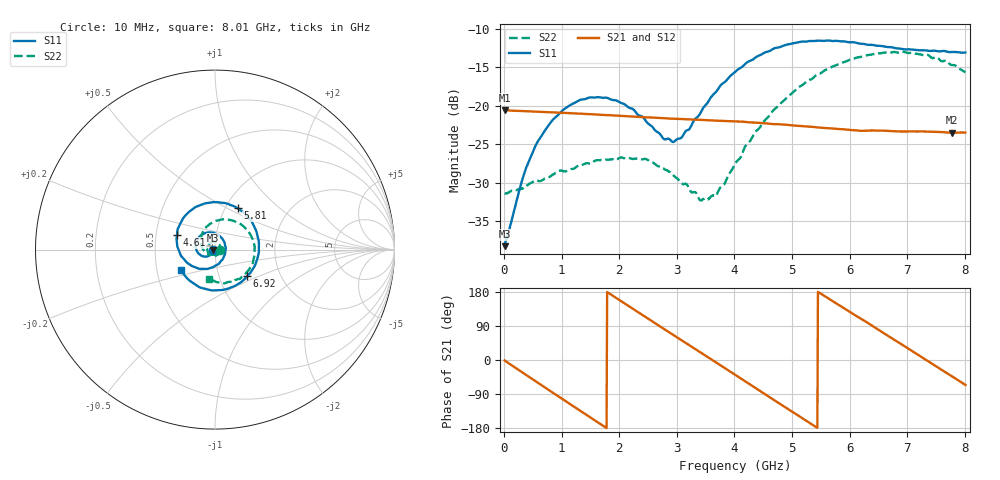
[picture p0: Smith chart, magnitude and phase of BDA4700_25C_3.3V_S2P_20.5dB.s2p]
!Agilent Technologies,E5071B,MY42404982,A.09.10
!Date: Mon Oct 20 18:11:40 2025
!Data & Calibration Information:
!Freq	S11:SOLT2(ON)	S21:SOLT2(ON)	S12:SOLT2(ON)	S22:SOLT2(ON)
# Hz S RI R 50
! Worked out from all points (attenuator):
!   801 points, 10 MHz to 8.01 GHz, reference 50 ohm
!   highest |S21| = -20.58 dB at 10 MHz (marker M1); lowest = -23.5 dB at 7.78 GHz (marker M2)
!   lowest |S11| = -38.3 dB at 10 MHz (marker M3), VSWR 1.02, Z = 48.8 - j0.152 ohm
!   |S11| at or under -10 dB: start of sweep to end of sweep
!   |S22| runs from -32.3 to -13.0 dB; largest |S21 - S12| = 0.0011
!   S11 on the Smith chart (normalised r, x): 10 MHz: 0.98, -0.00; 4.61 GHz: 0.64, +0.11; 5.81 GHz: 1.14, +0.56; 6.92 GHz: 1.36, -0.43; 8.01 GHz: 0.67, -0.16
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1e7  -0.0121 -0.00155  0.0936 -0.00201  0.0935 -0.0021  0.0269 -0.000806
3.4e8  -0.0231 -0.0266  0.0755 -0.0528  0.0755 -0.0529  0.0232 -0.018
5.7e8  -0.0424 -0.0383  0.0481 -0.0778  0.0481 -0.0778  0.0148 -0.0291
8.7e8  -0.0751 -0.0342  0.0023 -0.0904  0.00241 -0.0904  -0.00639 -0.0355
1.35e9  -0.1083 0.0177  -0.0645 -0.0608  -0.0645 -0.0608  -0.037 -0.018
1.97e9  -0.0547 0.0924  -0.0817 0.0274  -0.0817 0.0274  -0.0345 0.0288
2.45e9  0.0245 0.077  -0.0343 0.0767  -0.0344 0.0768  -0.00217 0.0452
2.68e9  0.0516 0.0425  -0.00215 0.0833  -0.00229 0.0833  0.0142 0.0378
2.96e9  0.0572 -0.0127  0.0358 0.074  0.0358 0.0738  0.0269 0.0221
3.43e9  -0.00201 -0.0928  0.0769 0.0252  0.0769 0.0252  0.0197 -0.0142
3.69e9  -0.0629 -0.1071  0.0793 -0.0101  0.0794 -0.0103  0.000595 -0.0263
4.01e9  -0.1441 -0.0809  0.0617 -0.0496  0.0618 -0.0495  -0.0323 -0.0263
4.61e9  -0.2113 0.0819  -0.0107 -0.0756  -0.0104 -0.0757  -0.0787 0.0362
4.95e9  -0.1673 0.1871  -0.0494 -0.0563  -0.0493 -0.0566  -0.0702 0.0925
5.35e9  -0.0437 0.2594  -0.0718 -0.0121  -0.0717 -0.0126  -0.0154 0.1487
5.81e9  0.1256 0.2311  -0.0581 0.0401  -0.0579 0.0402  0.0875 0.1644
6.25e9  0.2314 0.0995  -0.0167 0.0666  -0.0157 0.0668  0.1819 0.1046
6.68e9  0.2302 -0.0687  0.0318 0.0607  0.0318 0.0607  0.2201 -0.0022
6.92e9  0.1795 -0.1488  0.0523 0.0434  0.0524 0.043  0.2125 -0.0699
7.34e9  0.0333 -0.2257  0.0679 -0.00108  0.0679 -0.00106  0.1409 -0.1609
7.78e9  -0.1327 -0.1796  0.0484 -0.0458  0.0483 -0.046  0.0221 -0.1823
8.01e9  -0.1896 -0.1148  0.0273 -0.0611  0.0276 -0.061  -0.0325 -0.1612
